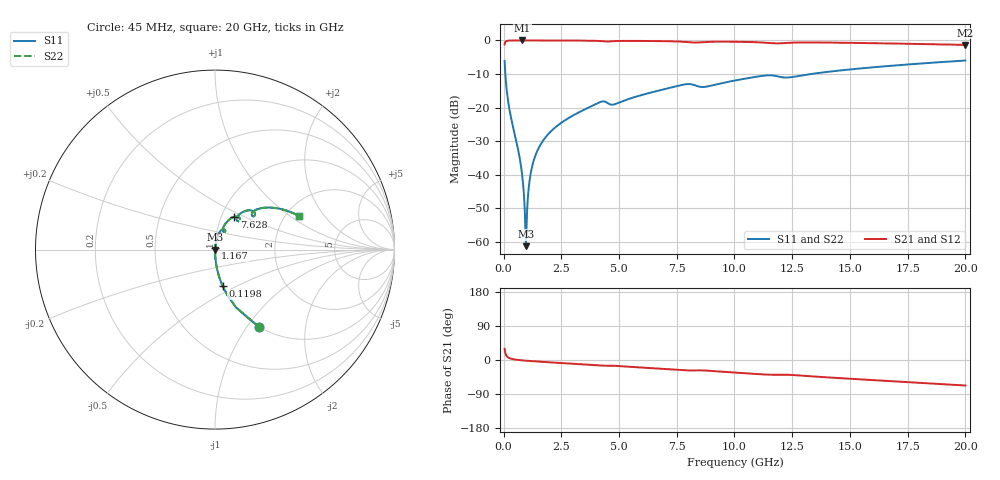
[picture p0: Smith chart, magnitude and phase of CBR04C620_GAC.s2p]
! S-parameter model data by Modelithics Inc.  support@modelithics.com 813-866-6335  Tampa FL USA
! S-Parameter data specifications:
! Substrate: 20-mil Rogers 4350B, substrate thickness, H=0.508mm, Dielectric constant, Er=3.75
! PCB Mounting Pad Footprint: Pad width, PadW=0.52mm , Pad length, PadL=0.52mm , Pad gap, PadG (edge-to-edge)=0.28mm , Reference planes=1.32mm apart
#  GHz  S  MA  R 50
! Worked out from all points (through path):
!   801 points, 45 MHz to 20 GHz, reference 50 ohm
!   highest |S21| = -0.01 dB at 818.3 MHz (marker M1); lowest = -1.3 dB at 20 GHz (marker M2)
!   group delay of S21, straight-line fit = 9.47 ps
!   lowest |S11| = -61.3 dB at 967.9 MHz (marker M3), VSWR 1.00, Z = 50.1 - j0.00036 ohm
!   |S11| at or under -10 dB: 77.01 MHz to 13.33 GHz (13.25 GHz wide, 198 % of centre)
!   |S22| runs from -61.3 to -6.0 dB; largest |S21 - S12| = 0
!   S11 on the Smith chart (normalised r, x): 45 MHz: 1.00, -1.14; 119.8 MHz: 1.00, -0.42; 1.167 GHz: 1.00, +0.02; 7.628 GHz: 1.15, +0.44; 20 GHz: 2.33, +1.17
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0.045  0.4941 -60.5  0.8692 29.5  0.8692 29.5  0.4941 -60.5
0.119831  0.2061 -78.2  0.9782 11.7  0.9782 11.7  0.2061 -78.2
0.294438  0.07874 -85.7  0.9964 4.0  0.9964 4.0  0.07874 -85.7
0.668594  0.02005 -88.1  0.9991 -0.1  0.9991 -0.1  0.02005 -88.1
0.818256  0.008963 -86.0  0.9991 -1.0  0.9991 -1.0  0.008963 -86.0
0.893088  0.00433 -80.5  0.9991 -1.4  0.9991 -1.4  0.00433 -80.5
0.967919  0.000857 -0.2  0.9991 -1.8  0.9991 -1.8  0.000857 -0.2
1.04275  0.00408 75.2  0.9991 -2.2  0.9991 -2.2  0.00408 75.2
1.167469  0.01009 81.9  0.999 -2.7  0.999 -2.7  0.01009 81.9
1.416906  0.02083 83.3  0.9987 -3.8  0.9987 -3.8  0.02083 83.3
1.816006  0.03591 82.7  0.9981 -5.4  0.9981 -5.4  0.03591 82.7
2.4396  0.05722 80.7  0.9968 -7.8  0.9968 -7.8  0.05722 80.7
3.387462  0.08902 77.0  0.9935 -11.4  0.9935 -11.4  0.08902 77.0
4.23555  0.1222 67.6  0.9764 -14.8  0.9764 -14.8  0.1222 67.6
4.784313  0.1112 66.0  0.9766 -15.2  0.9766 -15.2  0.1112 66.0
6.704981  0.1784 65.5  0.978 -22.7  0.978 -22.7  0.1784 65.5
7.6279  0.2136 59.5  0.9615 -26.4  0.9615 -26.4  0.2136 59.5
8.700481  0.2028 53.2  0.9471 -27.7  0.9471 -27.7  0.2028 53.2
10.0225  0.2528 54.3  0.9561 -33.2  0.9561 -33.2  0.2528 54.3
13.36496  0.3176 44.2  0.9339 -43.2  0.9339 -43.2  0.3176 44.2
16.68248  0.4163 33.6  0.902 -55.5  0.902 -55.5  0.4163 33.6
20  0.5021 22.0  0.858 -67.3  0.858 -67.3  0.5021 22.0
